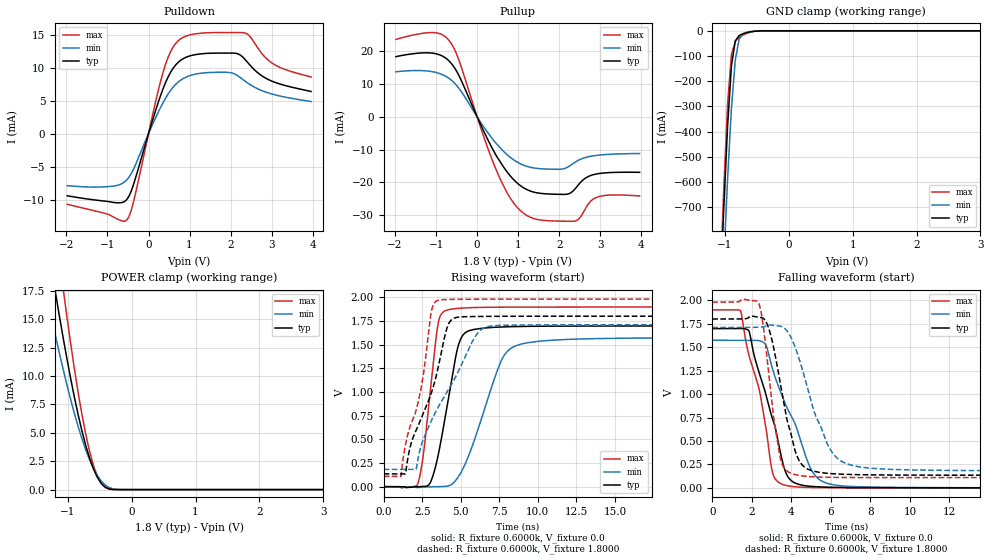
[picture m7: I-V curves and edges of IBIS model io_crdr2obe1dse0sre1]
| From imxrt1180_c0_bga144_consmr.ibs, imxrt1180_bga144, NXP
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[Model]  io_crdr2obe1dse0sre1
|   Model io_crdr2obe1dse0sre1
| This model was characterised for following simulation conditions:
| External (pad) voltage:
|   - Typ: 1.8V,   - Min: 1.71V,   - Max: 1.98V
| Library cells for typ/min/max conditions are connected as defined below:
|  PAD_IO - External Pad
|  ipp_do - Core Input
|  ipp_obe - Output Buffer Enable
|  ASRCN3V3[3] - NC
|  ASRCN3V3[4] - NC
|  ASRCP3V3[4] - NC
|  REFAPBIAS3V3 - gnde
|  REFBAMPL3V3 - vdd1v8
|  REFCAMPH3V3 - vdd1v8
|  REFDNBIAS3V3 - vdd1v8
|  REFH3V3 - REFH3V3
|  REFL3V3 - REFL3V3
|  gnde - gnde
|  ipp_dse - gnde
|  ipp_ina235_3v - NC
|  ipp_ina40_3v - NC
|  ipp_ina_mux - NC
|  ipp_ind - NC
|  ipp_ind_1p8v - NC
|  ipp_ind_3v - NC
|  ipp_sre - vdd
|  vdd - vdd
|  vdd1v8 - vdd1v8
|  vdda - vdde3v3
|  vdde3v3 - vdde3v3
| All other pins connected to ground
Model_type I/O
Polarity   Non-Inverting
Enable   Active-High
Vinl =   0.5400V
Vinh =   1.2600V
Vmeas =  0.9000V
Cref =   15.0000pF
Rref =   0.6000k
Vref =   0.0V
C_comp   3.9792pF   3.7942pF   4.1043pF
|C_comp_pullup   0.4867pF   0.5822pF   0.4755pF
|C_comp_pulldown   2.0823pF   2.1675pF   1.8519pF
[Model Spec]
| variable   typ   min   max
Vinh   1.2600V   NA   NA
Vinl   0.5400V   NA   NA
Vref   0.0V   0.0V   0.0V
Cref   15.0000pF   15.0000pF   15.0000pF
Rref   0.6000k   0.6000k   0.6000k
[Receiver Thresholds]
Vcross_high  =   0.0V
Vcross_low  =   0.0V
Vdiff_ac  =   0.0V
Vdiff_dc  =   0.0V
Tdiffslew_ac  =   0.0S
[Temperature Range]   25.0000   0.1250k   -40.0000
[Voltage Range]   1.8000V   1.7100V   1.9800V
[Pullup Reference]   1.8000V   1.7100V   1.9800V
[Pulldown Reference]   0.0V   0.0V   0.0V
[POWER Clamp Reference]   1.8000V   1.7100V   1.9800V
[GND Clamp Reference]   0.0V   0.0V   0.0V
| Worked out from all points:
|   slope of the pulldown table from 0 to 0.27 V, typ, clamps not added: 50.4 ohm
|   slope of the pullup table from 0 to 0.27 V, typ, clamps not added: 37.4 ohm
|   GND clamp passes 1 mA (typ) near -0.50 V on its own axis
|   POWER clamp passes 1 mA (typ) near -0.53 V on its own axis
|   rising waveform, R_fixture 0.6000k, V_fixture 0.0: 20-80 % time 1.11ns typ, 1.96ns min, 754ps max; typ from 0 V to 1.7 V
|   rising waveform, R_fixture 0.6000k, V_fixture 1.8000: 20-80 % time 2ns typ, 2.83ns min, 1.43ns max; typ from 0.135 V to 1.8 V
|   falling waveform, R_fixture 0.6000k, V_fixture 0.0: 20-80 % time 1.3ns typ, 1.7ns min, 1.14ns max; typ from 1.7 V to 0 V
|   falling waveform, R_fixture 0.6000k, V_fixture 1.8000: 20-80 % time 965ps typ, 1.43ns min, 655ps max; typ from 1.8 V to 0.135 V
[Pulldown]
|Voltage   I(typ)   I(min)   I(max)
-1.98V    -9.436mA   -7.894mA   -10.73mA
-840mV    -10.46mA   -7.944mA   -12.69mA
-600mV    -10.36mA   -7.4mA     -13.31mA
-480mV    -9.54mA    -6.639mA   -12.65mA
-360mV    -7.618mA   -5.325mA   -10.21mA
360mV     6.913mA    4.777mA    9.448mA
600mV     9.943mA    7.063mA    13.16mA
840mV     11.38mA    8.355mA    14.62mA
1.92V     12.24mA    9.317mA    15.36mA
2.34V     11.36mA    8.04mA     15.32mA
3V        7.996mA    6.036mA    10.77mA
3.96V     6.411mA    4.879mA    8.598mA
[Pullup]
|Voltage   I(typ)   I(min)   I(max)
-1.98V    18.38mA    13.75mA    23.61mA
-1.08V    19.43mA    13.76mA    25.73mA
-660mV    16.76mA    11.5mA     22.93mA
-420mV    12.02mA    8.321mA    16.48mA
180mV     -4.905mA   -3.419mA   -6.743mA
540mV     -13.3mA    -9.177mA   -18.38mA
840mV     -18.52mA   -12.69mA   -25.44mA
1.2V      -22.16mA   -15.08mA   -30.05mA
2.04V     -23.69mA   -16.02mA   -31.87mA
2.4V      -21.82mA   -13.76mA   -31.82mA
2.94V     -17.39mA   -11.74mA   -24.47mA
3.96V     -16.96mA   -11.21mA   -24.17mA
[GND_clamp]
|Voltage   I(typ)   I(min)   I(max)
-1.98V    -7.543A    -7.6A      -7.897A
-1.08V    -1.077A    -1.286A    -1.025A
-1.02V    -705.3mA   -921.3mA   -628.8mA
-960mV    -377.1mA   -587.4mA   -291.7mA
-900mV    -139.2mA   -307mA     -94.38mA
-840mV    -40.12mA   -117mA     -42.82mA
-780mV    -18.81mA   -33.95mA   -26.13mA
-720mV    -11.86mA   -11.44mA   -16.78mA
-660mV    -7.061mA   -5.737mA   -9.992mA
-540mV    -1.684mA   -1.901mA   -2.15mA
-420mV    -207.1uA   -403.7uA   -160.6uA
3.96V     0A         0A         0A
[POWER_clamp]
|Voltage   I(typ)   I(min)   I(max)
-1.98V    46.79mA    35.94mA    61.38mA
-1.32V    21.77mA    16.85mA    28.91mA
-1.2V     17.57mA    13.71mA    23.33mA
-1.14V    15.55mA    12.2mA     20.62mA
-1.08V    13.59mA    10.75mA    17.99mA
-1.02V    11.7mA     9.353mA    15.46mA
-900mV    8.209mA    6.76mA     10.73mA
-720mV    3.898mA    3.51mA     4.887mA
-540mV    1.103mA    1.267mA    1.195mA
-420mV    244.5uA    429.2uA    190.6uA
-180mV    280.9nA    5.273uA    26.8nA
3.96V     0A         0A         0A
[Ramp]
| variable   typ   min   max
dV/dt_r  1.0186/1.1125n   0.9439/1.9603n   1.1383/0.7540n
dV/dt_f  0.9990/0.9653n   0.9166/1.4305n   1.1224/0.6554n
R_load = 0.6000k
[Rising Waveform]
R_fixture= 0.6000k
V_fixture= 0.0
V_fixture_min= 0.0
V_fixture_max= 0.0
|time   V(typ)   V(min)   V(max)
0s        115.1nV    3.181uV    43.69nV
2.219ns   -2.115mV   -8.074mV   34.42mV
2.983ns   30.75mV    -1.873mV   948mV
3.527ns   325.8mV    -310.6uV   1.718V
4.275ns   1.006V     12.14mV    1.871V
4.789ns   1.46V      91.6mV     1.882V
5.254ns   1.62V      227.6mV    1.887V
7.642ns   1.686V     1.336V     1.895V
9.206ns   1.692V     1.515V     1.896V
60ns      1.698V     1.573V     1.897V
[Rising Waveform]
R_fixture= 0.6000k
V_fixture= 1.8000
V_fixture_min= 1.7100
V_fixture_max= 1.9800
|time   V(typ)   V(min)   V(max)
0s        135mV      182.4mV    109.3mV
1.117ns   134.1mV    182.3mV    109.1mV
1.416ns   137.6mV    181.8mV    443.9mV
2.103ns   592.6mV    185.2mV    806.8mV
3.094ns   990.7mV    697.7mV    1.849V
3.589ns   1.3V       855.1mV    1.97V
4.408ns   1.764V     1.082V     1.977V
6.015ns   1.797V     1.603V     1.979V
7.085ns   1.798V     1.698V     1.98V
60ns      1.8V       1.71V      1.98V
[Falling Waveform]
R_fixture= 0.6000k
V_fixture= 0.0
V_fixture_min= 0.0
V_fixture_max= 0.0
|time   V(typ)   V(min)   V(max)
0s        1.698V     1.573V     1.897V
1.418ns   1.699V     1.573V     1.891V
1.848ns   1.675V     1.572V     1.418V
2.686ns   1.016V     1.532V     678.6mV
3.07ns    723.2mV    1.252V     148mV
3.617ns   226.9mV    936.1mV    32.75mV
3.976ns   80.64mV    773.5mV    16.33mV
5.177ns   13.11mV    138mV      3.006mV
6.784ns   3.808mV    17.4mV     504.9uV
60ns      7.064uV    14.69uV    3.067uV
[Falling Waveform]
R_fixture= 0.6000k
V_fixture= 1.8000
V_fixture_min= 1.7100
V_fixture_max= 1.9800
|time   V(typ)   V(min)   V(max)
0s        1.8V       1.71V      1.98V
2.341ns   1.82V      1.713V     1.974V
2.564ns   1.81V      1.715V     1.751V
2.851ns   1.704V     1.735V     1.226V
3.453ns   1.102V     1.722V     307.3mV
3.821ns   691.3mV    1.662V     173.8mV
4.473ns   263.6mV    1.321V     129.2mV
6.025ns   151.5mV    390.2mV    111.9mV
7.764ns   139.3mV    214.7mV    109.6mV
60ns      135mV      182.4mV    109.3mV
